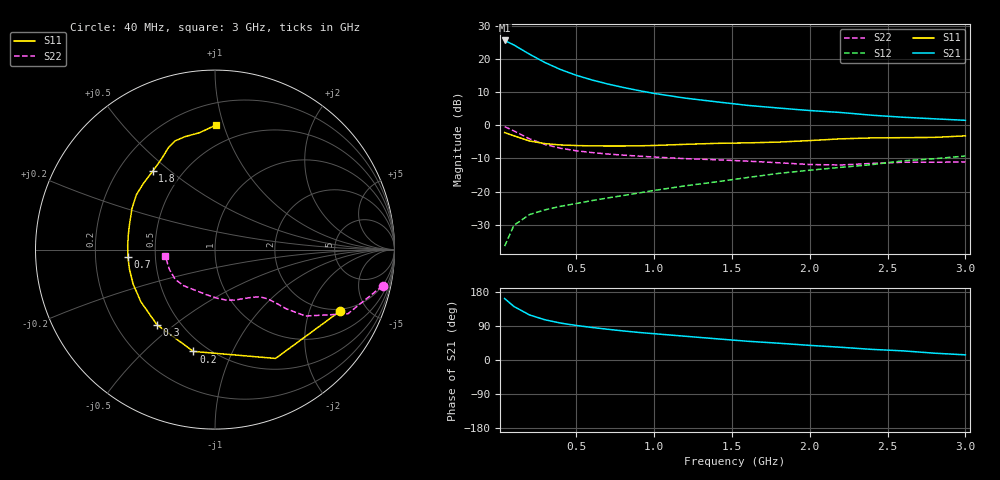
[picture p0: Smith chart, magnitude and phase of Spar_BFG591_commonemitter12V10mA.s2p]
! Filename:  BFG591A.S2P  Version:  4.0
! NXP part #: BFG591  Date: Jun 1994
! Bias condition: Vce=12V; Ic=10mA
#  MHz  S  MA  R  50
! Freq  S11  S21  S12  S22  !GUM [dB]
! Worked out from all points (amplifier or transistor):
!   21 points, 40 MHz to 3 GHz, reference 50 ohm
!   highest |S21| = 25.6 dB at 40 MHz (marker M1)
!   |S21| within 3 dB of that: start of sweep to 158.8 MHz
!   unconditionally stable (mu >= 1): 767.3 MHz to 2.161 GHz
!   at 300 MHz: K = 0.58, MSG = 22.2 dB, |S12| = -25.5 dB
!   at 1 GHz: K = 1.07, MAG = 13.0 dB, |S12| = -19.7 dB
!   at 3 GHz: K = 0.96, MSG = 5.4 dB, |S12| = -9.3 dB
!   S11 on the Smith chart (normalised r, x): 40 MHz: 1.89, -3.26; 200 MHz: 0.42, -0.72; 300 MHz: 0.37, -0.43; 700 MHz: 0.35, -0.04; 1.8 GHz: 0.34, +0.44; 3 GHz: 0.35, +0.94
40  0.776 -26.3  19.07 162.1  0.015 77.2  0.955 -12.2
100  0.694 -60.9  16.28 141.2  0.031 62.9  0.822 -25.8
200  0.58 -102.0  11.83 118.9  0.045 52.4  0.625 -36.3
300  0.529 -127.7  8.836 106.0  0.053 50.2  0.513 -39.8
400  0.505 -144.9  6.933 97.4  0.06 51.0  0.45 -41.3
500  0.495 -157.3  5.685 91.1  0.066 53.2  0.413 -42.6
600  0.489 -167.2  4.842 85.9  0.073 55.1  0.388 -44.1
700  0.487 -175.4  4.213 81.2  0.08 57.3  0.369 -45.9
800  0.487 177.2  3.737 76.8  0.087 59.2  0.355 -48.0
900  0.49 170.3  3.347 72.8  0.095 61.1  0.343 -50.6
1000  0.496 164.1  3.029 69.4  0.104 62.5  0.332 -53.6
1200  0.516 153.7  2.572 62.7  0.122 64.4  0.314 -60.7
1400  0.534 145.2  2.262 56.0  0.14 65.3  0.302 -68.8
1600  0.543 137.3  1.999 49.5  0.163 66.8  0.288 -77.5
1800  0.558 128.4  1.821 44.3  0.188 65.3  0.272 -87.0
2000  0.588 120.2  1.67 38.6  0.21 65.0  0.256 -100.4
2200  0.625 114.5  1.56 33.6  0.232 63.6  0.252 -116.1
2400  0.645 110.3  1.419 28.0  0.255 63.5  0.266 -130.7
2600  0.651 104.9  1.323 24.1  0.291 60.0  0.277 -143.2
2800  0.657 97.5  1.253 18.0  0.313 56.1  0.277 -156.3
3000  0.693 89.7  1.189 13.6  0.344 54.8  0.28 -172.8
